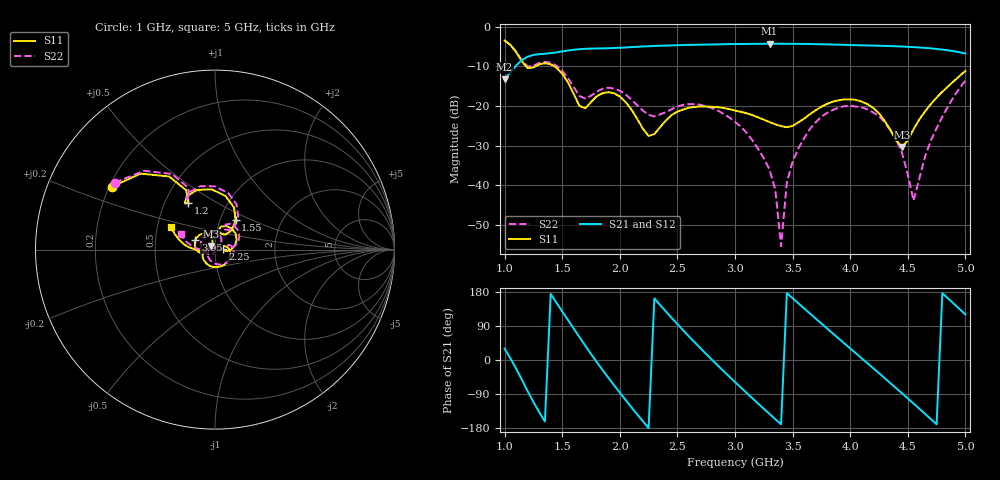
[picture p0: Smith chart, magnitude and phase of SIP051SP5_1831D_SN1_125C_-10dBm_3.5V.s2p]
# GHz  S  dB  R  50
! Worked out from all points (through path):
!   81 points, 1 GHz to 5 GHz, reference 50 ohm
!   highest |S21| = -4.25 dB at 3.3 GHz (marker M1); lowest = -13.2 dB at 1 GHz (marker M2)
!   lowest |S11| = -30.3 dB at 4.45 GHz (marker M3), VSWR 1.06, Z = 47.7 + j1.96 ohm
!   |S11| at or under -10 dB: 1.187 GHz to 1.265 GHz (78.01 MHz wide, 6.36 % of centre); 1.431 GHz to end of sweep
!   |S22| runs from -55.3 to -3.5 dB; largest |S21 - S12| = 0.0024
!   S11 on the Smith chart (normalised r, x): 1 GHz: 0.21, +0.27; 1.2 GHz: 0.66, +0.38; 1.55 GHz: 1.19, +0.40; 2.25 GHz: 1.09, +0.01; 3.95 GHz: 0.80, +0.09; 5 GHz: 0.59, +0.16
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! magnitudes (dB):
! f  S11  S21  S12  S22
! 1 GHz  -3.4  -13.2  -13.2  -3.5
! 1.2 GHz  -10.4  -7.5  -7.5  -10.0
! 1.4 GHz  -9.5  -6.6  -6.6  -9.1
! 1.55 GHz  -14.0  -6.0  -6.0  -12.9
! 1.7 GHz  -20.5  -5.5  -5.5  -18.1
! 1.95 GHz  -16.8  -5.3  -5.3  -15.6
! 2.25 GHz  -27.5  -4.9  -4.9  -22.2
! 2.35 GHz  -25.3  -4.8  -4.8  -22.1
! 2.65 GHz  -20.2  -4.5  -4.5  -19.5
! 3 GHz  -21.1  -4.3  -4.3  -24.0
! 3.3 GHz  -24.0  -4.3  -4.3  -36.1
! 3.35 GHz  -24.6  -4.3  -4.3  -41.1
! 3.4 GHz  -25.1  -4.3  -4.2  -55.3
! 3.45 GHz  -25.3  -4.3  -4.3  -39.2
! 3.5 GHz  -25.0  -4.3  -4.3  -34.0
! 3.7 GHz  -21.1  -4.4  -4.4  -24.1
! 3.95 GHz  -18.3  -4.5  -4.5  -20.0
! 4.35 GHz  -26.1  -4.9  -4.9  -26.2
! 4.45 GHz  -30.3  -5.0  -5.0  -31.8
! 4.55 GHz  -25.8  -5.1  -5.1  -43.8
! 4.7 GHz  -19.5  -5.4  -5.4  -28.7
! 5 GHz  -11.1  -6.7  -6.7  -13.6
